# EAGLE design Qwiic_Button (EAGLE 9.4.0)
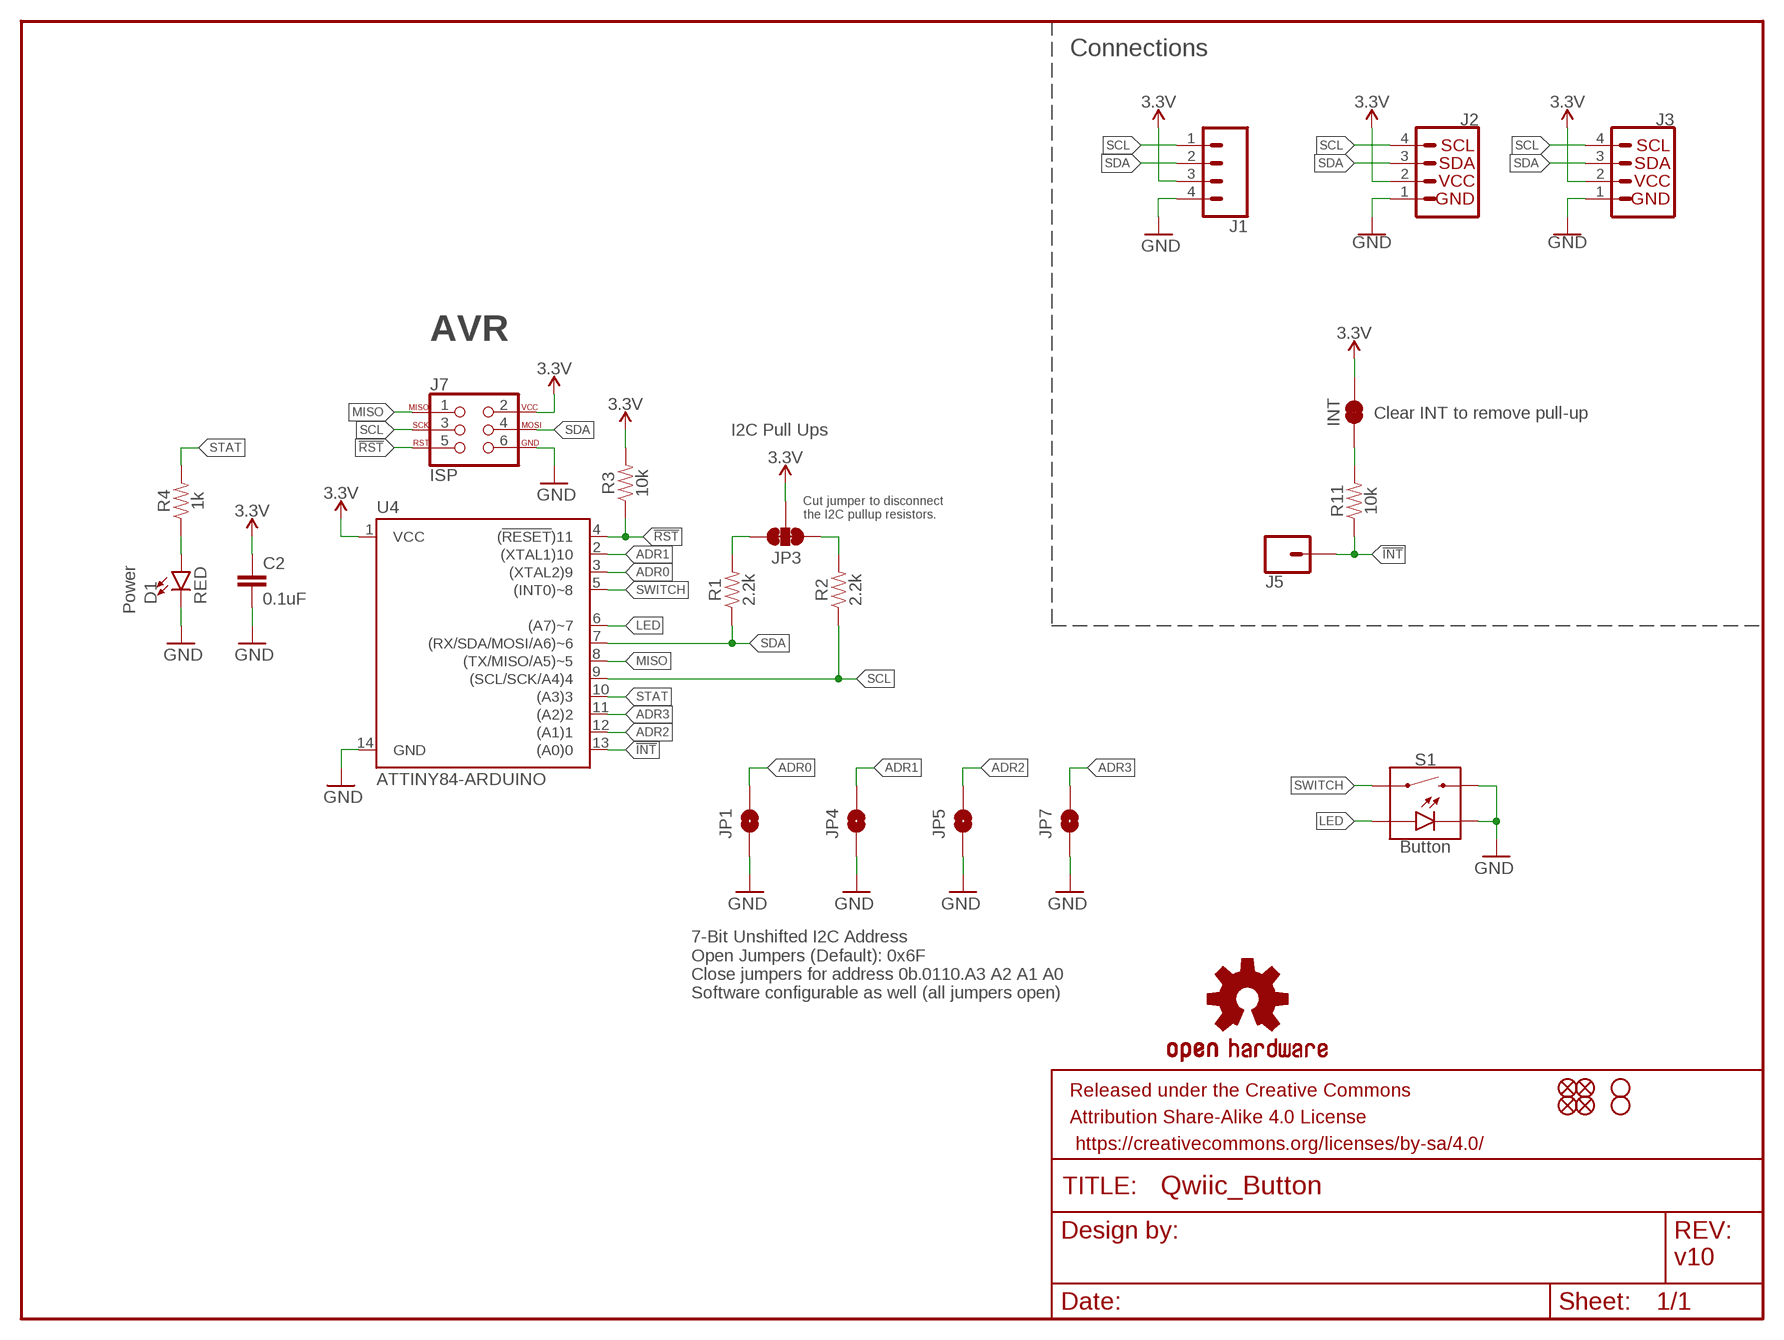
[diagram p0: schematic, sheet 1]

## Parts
C2  0.1uF  0.1UF-0603-25V-(+80/-20%)  [0603]
D1  RED  LED-RED0603  [LED-0603]
FRAME1  FRAME-LETTER  [CREATIVE_COMMONS]
H1  STAND-OFF  [STAND-OFF]
H2  STAND-OFF  [STAND-OFF]
INT  JUMPER-SMT_2_NC_TRACE_SILK  [SMT-JUMPER_2_NC_TRACE_SILK]
J1  CONN_041X04_NO_SILK  [1X04_NO_SILK]
J2  QWIIC_CONNECTORJS-1MM  [JST04_1MM_RA]
J3  QWIIC_CONNECTORJS-1MM  [JST04_1MM_RA]
J5  CONN_01PTH_NO_SILK_YES_STOP  [1X01_NO_SILK]
J7  ISP  AVR_SPI_PROG_3X2TESTPOINTS  [2X3_TEST_POINTS]
JP1  JUMPER-SMT_2_NO_SILK  [SMT-JUMPER_2_NO_SILK]
JP2  FIDUCIALUFIDUCIAL  [MICRO-FIDUCIAL]
JP3  JUMPER-SMT_3_2-NC_TRACE_SILK  [SMT-JUMPER_3_2-NC_TRACE_SILK]
JP4  JUMPER-SMT_2_NO_SILK  [SMT-JUMPER_2_NO_SILK]
JP5  JUMPER-SMT_2_NO_SILK  [SMT-JUMPER_2_NO_SILK]
JP6  FIDUCIALUFIDUCIAL  [MICRO-FIDUCIAL]
JP7  JUMPER-SMT_2_NO_SILK  [SMT-JUMPER_2_NO_SILK]
JP8  FIDUCIALUFIDUCIAL  [MICRO-FIDUCIAL]
JP9  FIDUCIALUFIDUCIAL  [MICRO-FIDUCIAL]
LOGO1  OSHW-LOGOMINI  [OSHW-LOGO-MINI]
R1  2.2k  2.2KOHM-0603-1/10W-1%  [0603]
R2  2.2k  2.2KOHM-0603-1/10W-1%  [0603]
R3  10k  10KOHM-0603-1/10W-1%  [0603]
R4  1k  1KOHM-0603-1/10W-1%  [0603]
R11  10k  10KOHM-0603-1/10W-1%  [0603]
S1  Button  MOMENTARY-SWITCH-SPST-LED-PTH-12MM  [TACTILE_SWITCH_LED_PTH_12MM]
U4  ATTINY84-ARDUINO  [SO14]

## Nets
3.3V: C2.1 INT.2 J1.3 J2.2 J3.2 J7.2 JP3.2 R3.2 U4.1(VCC)
!INT: J5.1 R11.1 U4.13((A0)0)
!RST: J7.5 R3.1 U4.4((!RESET!)11)
ADR0: JP1.2 U4.3((XTAL2)9)
ADR1: JP4.2 U4.2((XTAL1)10)
ADR2: JP5.2 U4.12((A1)1)
ADR3: JP7.2 U4.11((A2)2)
GND: C2.2 D1.C J1.4 J2.1 J3.1 J7.6 JP1.1 JP4.1 JP5.1 JP7.1 S1.2 S1.C U4.14(GND)
INT_R: INT.1 R11.2
LED: S1.A U4.6((A7)~7)
MISO: J7.1 U4.8((TX/MISO/A5)~5)
N$3: D1.A R4.1
SCL: J1.1 J2.4 J3.4 J7.3 R2.1 U4.9((SCL/SCK/A4)4)
SCL_PU1: JP3.1 R2.2
SDA: J1.2 J2.3 J3.3 J7.4 R1.1 U4.7((RX/SDA/MOSI/A6)~6)
SDA_PU1: JP3.3 R1.2
STAT: R4.2 U4.10((A3)3)
SWITCH: S1.4 U4.5((INT0)~8)

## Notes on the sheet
- Connections
- AVR
- Clear INT to remove pull-up
- I2C Pull Ups
- Cut jumper to disconnect
  the I2C pullup resistors.
- Power
- 7-Bit Unshifted I2C Address
  Open Jumpers (Default): 0x6F
  Close jumpers for address 0b.0110.A3 A2 A1 A0
  Software configurable as well (all jumpers open)
- v10

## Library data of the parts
C2 = SparkFun-Capacitors:0.1UF: 0.1µF ceramic capacitors; PROD_ID: CAP-00810
D1 = SparkFun-LED:LED-RED: Red SMD LED; PROD_ID: DIO-00819
FRAME1 = SparkFun-Aesthetics:FRAME-LETTER: Schematic Frame - Letter
H1 H2 = SparkFun-Hardware:STAND-OFF: Stand Off
INT = SparkFun-Jumpers:JUMPER-SMT_2_NC_TRACE: Normally closed trace jumper
J1 = SparkFun-Connectors:CONN_04: Multi connection point. Often used as Generic Header-pin footprint for 0.1 inch spaced/style header connections On any of the 0.1 inch spaced packages, you can populate with these: Break Away Headers - Straight (PRT-00116) Break Away Male Headers - Right Angle (PRT-00553) Female Headers (PRT-00115)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; PROD_ID: CONN-09696
J2 J3 = SparkFun-Connectors:QWIIC_CONNECTOR: SparkFun I2C Standard Qwiic Connector An SMD 1mm pitch JST connector makes it easy and quick (get it? Qwiic?) to connect I2C devices to each other. The Qwiic system enables fast and solderless connection between popular platforms and various sensors and actuators. We carry 200mm, 100mm, 50mm, and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; PROD_ID: CONN-13694
J5 = SparkFun-Connectors:CONN_01: Single connection point. Often used as Generic Header-pin footprint for 0.1 inch spaced/style header connections
J7 = SparkFun-Connectors:AVR_SPI_PROG_3X2: AVR ISP 6 Pin This is the reduced ISP connector for AVR programming. Common on Arduino. This footprint will take up less PCB space and can be used with a 10-pin to 6-pin adapter such as SKU: BOB-08508 **Special note about "TEST_POINT" package. The stop mask is on the top side, so if you want your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
JP1 JP4 JP5 JP7 = SparkFun-Jumpers:JUMPER-SMT_2_NO: Normally open jumper
JP2 JP6 JP8 JP9 = SparkFun:FIDUCIAL: Fiducial Alignment Points
JP3 = SparkFun-Jumpers:JUMPER-SMT_3_2-NC_TRACE: Normally closed trace jumper (2 of 2 connections) This jumper has a trace between all three pads so they are normally closed (NC). Use a razor knife to open the connection(s). For best results follow the IPC guidelines for cutting traces: Cutout at least 0.063 mm (0.005 in). Remove all loose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
LOGO1 = SparkFun-Aesthetics:OSHW-LOGO: Open-Source Hardware (OSHW) Logo
R1 R2 = SparkFun-Resistors:2.2KOHM: 2.2kΩ resistor; PROD_ID: RES-08272
R3 R11 = SparkFun-Resistors:10KOHM: 10kΩ resistor; PROD_ID: RES-00824
R4 = SparkFun-Resistors:1KOHM: 1kΩ resistor; PROD_ID: RES-07856
S1 = SparkFun-Switches:MOMENTARY-SWITCH-SPST-LED: Momentary Switch (Pushbutton) - SPST - w/ LED Normally-open (NO) SPST momentary switches (buttons, pushbuttons), with a built-in LED. Variants PTH-CHERRY - Cherry MX Switch Cherry MX Keyswitches are top-of-the-line mechanical keyboard switches. They’re satisfyingly “clicky”, reliable up to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; PROD_ID: SWCH-11758; SF_SKU: COM-10442
U4 = SparkFun-IC-Microcontroller:ATTINY84-ARDUINO; PROD_ID: IC-14155

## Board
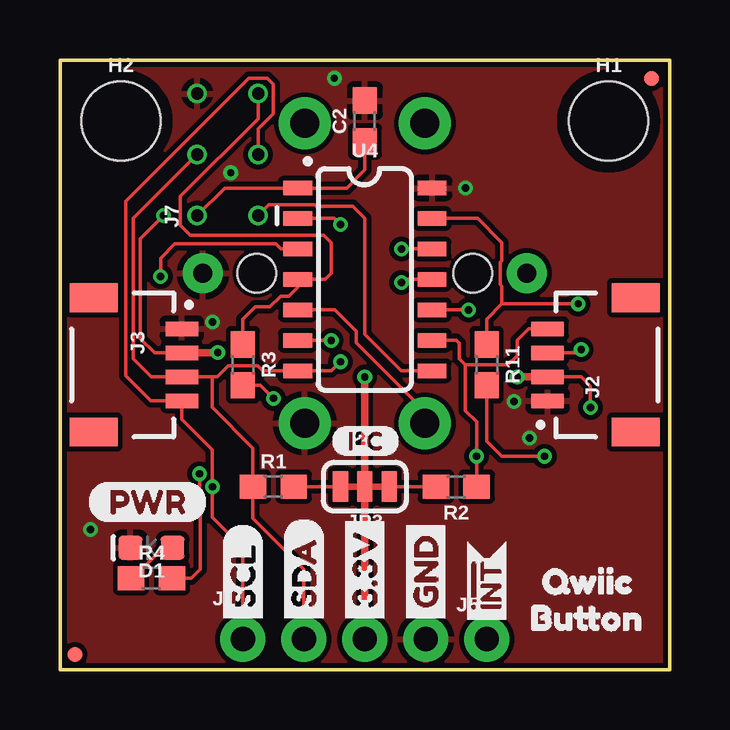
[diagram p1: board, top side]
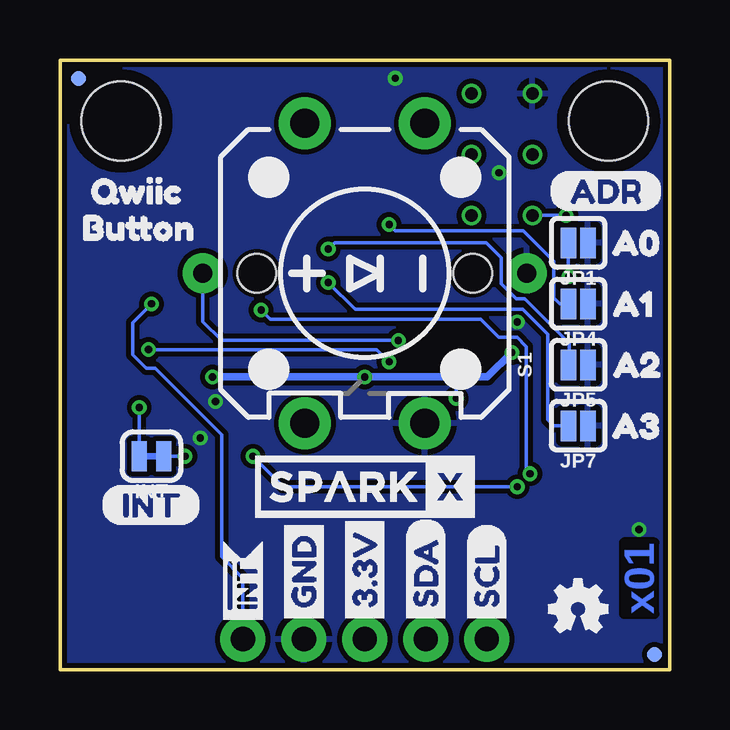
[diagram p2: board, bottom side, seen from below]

Size 25.4 x 25.4 mm. Coordinates in mm from the lower left corner, seen from the top.
Outline: 0,0 25.4,0 25.4,25.4 0,25.4 0,0
Copper layers (1*16): Top 0.035mm / dielectric 1.5mm / Bottom 0.035mm
Design rules "SparkFun-2-layer-PCBWay-LIMIT": minimum track width 6mil, minimum drill 0.3mm, track to track 6mil, track to pad 6mil, pad to pad 6mil, via to via 6mil, smd to smd 6mil, copper to edge 6mil, drill to drill 6mil, minimum pad ring 6mil, minimum via ring 6mil, stop-mask expansion 4mil, vias tented up to drill 25mil, thermal gap 10mil

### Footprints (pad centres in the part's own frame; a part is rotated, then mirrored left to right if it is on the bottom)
0603 = smd 1.1 x 1: 1 -0.85,0; 2 0.85,0
LED-0603 = smd 1 x 1: A -0.877,0; C 0.877,0
STAND-OFF = hole 3.302: 0,0
SMT-JUMPER_2_NC_TRACE_SILK = smd 0.635 x 1.27: 1 -0.508,0; 2 0.508,0
1X04_NO_SILK = drill 1.016 pad 1.88: 1 0,0; 2 2.54,0; 3 5.08,0; 4 7.62,0
JST04_1MM_RA = smd 0.6 x 1.35: 1 -1.5,0; 2 -0.5,0; 3 0.5,0; 4 1.5,0 | smd 1.2 x 2: NC1 2.8,-3.675; NC2 -2.8,-3.675
1X01_NO_SILK = drill 1.016 pad 1.88: 1 0,0
2X3_TEST_POINTS = drill 0.508: 1 -2.54,-1.27; 2 -2.54,1.27; 3 0,-1.27; 4 0,1.27; 5 2.54,-1.27; 6 2.54,1.27
SMT-JUMPER_2_NO_SILK = smd 0.635 x 1.27: 1 -0.406,0; 2 0.406,0
MICRO-FIDUCIAL = smd 0.635 x 0.635: 1 0,0
SMT-JUMPER_3_2-NC_TRACE_SILK = smd 0.635 x 1.27: 1 -1.016,0; 2 0,0; 3 1.016,0
TACTILE_SWITCH_LED_PTH_12MM = drill 1.2 pad 2.159: 1 -6.25,2.5; 2 6.25,2.5; 3 -6.25,-2.5; 4 6.25,-2.5 | drill 0.8 pad 1.676: A 0,-6.75; C 0,6.75 | hole 1.6: 0,4.5; 0,-4.5
SO14 = smd 0.6 x 1.2: 1 -3.175,-2.8; 2 -1.905,-2.8; 3 -0.635,-2.8; 4 0.635,-2.8; 5 1.905,-2.8; 6 3.175,-2.8; 7 4.445,-2.8; 8 4.445,2.8; 9 3.175,2.8; 10 1.905,2.8; 11 0.635,2.8; 12 -0.635,2.8; 13 -1.905,2.8; 14 -3.175,2.8

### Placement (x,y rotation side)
C2  12.7,22.86 90 top
D1  3.81,5.08 180 top
FRAME1  not placed on the board
H1  22.86,22.86 0 top
H2  2.54,22.86 0 top
INT  21.59,8.89 180 bottom
J1  7.62,1.27 0 top
J2  20.32,12.7 90 top
J3  5.08,12.7 270 top
J5  17.78,1.27 0 top
J7  6.99,21.46 90 top
JP1  3.81,17.78 180 bottom
JP2  24.64,24.64 0 bottom
JP3  12.7,7.62 180 top
JP4  3.81,15.24 180 bottom
JP5  3.81,12.7 180 bottom
JP6  0.64,0.64 0 bottom
JP7  3.81,10.16 180 bottom
JP8  0.64,0.64 0 top
JP9  24.64,24.64 0 top
LOGO1  3.81,2.54 0 bottom
R1  8.89,7.62 0 top
R2  16.51,7.62 180 top
R3  7.62,12.7 270 top
R4  3.81,3.81 0 top
R11  17.78,12.7 270 top
S1  12.7,16.51 270 bottom
U4  12.7,16.89 270 top
U$1  [BUTTON1]  18.67,2.16 0 top
U$2  [BUTTON1]  25.4,18.41 0 bottom
U$3  [PWR-()-04]  1.14,6.99 0 top
U$4  [INT-()-04]  23.75,6.86 0 bottom
U$5  [SCL]  7.62,1.65 90 bottom
U$6  [SDA]  10.16,1.65 90 bottom
U$7  [3.3V]  12.7,1.65 90 bottom
U$8  [GND]  15.24,1.65 90 bottom
U$9  [(ADR)]  5.08,19.94 0 bottom
U$10  [I_SUPER2_C-()-03]  11.3,9.53 0 top
U$11  [INT#-[<-04]  17.78,1.4 90 top
U$12  [SDA]  10.16,1.65 90 top
U$13  [GND]  15.24,1.65 90 top
U$14  [SCL]  7.62,1.65 90 top
U$15  [INT#-[<-04]  17.78,1.4 90 bottom
U$16  [A00]  3.3,17.78 0 bottom
U$17  [A11]  3.43,15.24 0 bottom
U$18  [SPARKX-MEDIUM]  12.7,7.62 0 bottom
U$19  [A22]  3.43,12.7 0 bottom
U$20  [QWIIC0]  25.02,19.94 0 bottom
U$21  [A33]  3.3,10.16 0 bottom
U$22  [3.3V]  12.7,1.65 90 top
U$23  [QWIIC0]  19.18,3.68 0 top

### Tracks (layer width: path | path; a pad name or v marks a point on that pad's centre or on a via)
3.3V  (via drill 0.3)
  Top 0.152: J7.2 6.86,20.07 U4.1 11.94,20.07 12.7,20.83 C2.1 | v19.06,12.2 v19.05,12.19 | v6.57,13.21 v6.57,13.2 | R3.2 8.34,11.85 v8.89,11.3 | v22.1,10.92 22.1,11.81 21.71,12.2 J2.2 | J3.2 3.94,13.2 3.35,13.79 3.35,17.96 v4.32,18.92
  Top 0.305: J2.2 v19.06,12.2 | v6.57,13.2 J3.2 | v12.7,12.19 JP3.2 J1.3
  Bottom 0.152: v8.89,11.3 8.89,12.19 | INT.2 v22.1,10.92 | J7.2 v4.32,18.92
  Bottom 0.305: v19.05,12.19 v12.7,12.19 8.89,12.19 7.59,12.19 v6.57,13.21
!INT  (via drill 0.3)
  Top 0.152: U4.13 17.4,18.8 18.41,17.78 18.41,17.04 18.34,16.97 18.34,16.05 18.41,15.98 18.41,15.24 | 18.41,15.24 17.78,14.61 R11.1 | v21.59,15.24 18.41,15.24
  Bottom 0.152: J5.1 17.78,3.81 18.67,4.7 18.67,9.78 21.44,12.55 21.81,12.55 22.38,13.11 22.38,14.45 v21.59,15.23 v21.59,15.24
!RST
  Top 0.152: J7.5 8.26,22.96 5.02,19.72 5.02,18.51 5.43,18.09 10.99,18.09 11.3,17.78 11.3,16.51 11.05,16.26 U4.4 | U4.4 | R3.1 7.62,14.61 8.13,15.11 8.75,15.11 9.19,15.55 9.53,15.55 9.91,15.93 U4.4
ADR0  (via drill 0.3)
  Top 0.152: v4.19,16.38 4.19,17.14 4.79,17.74 8.98,17.74 9.2,17.53 U4.3
  Bottom 0.152: JP1.2 4.22,16.41 v4.19,16.38
ADR1  (via drill 0.3)
  Top 0.152: U4.2 11.43,18.8 v11.68,18.54
  Bottom 0.152: v11.68,18.54 11.43,18.29 6.1,18.29 4.83,17.02 4.83,15.49 4.57,15.24 JP4.2
ADR2  (via drill 0.3)
  Top 0.152: U4.12 v14.22,17.53
  Bottom 0.152: v14.22,17.53 13.96,17.79 7.65,17.79 7.02,17.16 7.02,16.07 6.39,15.44 6.04,15.44 4.19,13.59 4.19,12.72 JP5.2
ADR3  (via drill 0.3)
  Top 0.152: U4.11 14.35,16.26 v14.22,16.13
  Bottom 0.152: v14.22,16.13 13.11,15.01 6.12,15.01 5.08,13.97 5.08,10.41 4.83,10.16 JP7.2
GND  (via drill 0.3)
  other vias: 1.27,5.84 18.92,11.18 19.56,9.65 16.89,20.07 11.43,24.64 6.35,14.48 7.11,20.7
  pour Top (isolate 0.203): 0,0 0,25.4 25.4,25.4 25.4,0
  pour Bottom (isolate 0.203): 0,0 25.4,0 25.4,25.4 0,25.4
INT_R  (via drill 0.3)
  Top 0.152: R11.2 17.78,9.53 18.41,8.89 v20.19,8.89
  Bottom 0.152: v20.19,8.89 INT.1
LED  (via drill 0.3)
  Top 0.152: U4.6 v11.3,13.72
  Bottom 0.152: v11.3,13.72 18.67,13.72 19.45,14.5 S1.A
MISO
  Top 0.152: J7.1 8.7,19.36 10.61,19.36 10.67,19.3 12.19,19.3 12.7,18.8 12.7,13.97 14.22,12.45 U4.8
N$3
  Top 0.152: R4.1 3.04,3.81 4.31,5.08 D1.A
SCL  (via drill 0.3)
  Top 0.152: U4.9 16.51,13.72 16.64,13.59 16.64,12.95 16.89,12.7 | 16.89,12.7 18.66,12.7 18.79,12.83 18.8,12.83 19.05,13.08 19.05,13.72 19.53,14.2 J2.4 | R2.1 v17.36,8.89 17.36,10.33 16.89,10.79 16.89,12.7 | J1.1 7.62,5.08 6.35,6.35 v6.35,7.62 6.35,9.17 5.08,10.44 J3.4 3.79,11.2 2.74,12.24 2.74,19.52 7.87,24.64 8.64,24.64 8.89,24.39 8.89,23.16 8.26,22.53 J7.3
  Bottom 0.152: v6.35,7.62 16.09,7.62 v17.36,8.89
SCL_PU1
  Top 0.152: JP3.1 R2.2
SDA  (via drill 0.3)
  Top 0.152: J7.4 3.05,18.8 3.05,12.95 3.8,12.2 J3.3 6.35,12.2 | 6.35,12.2 6.54,12.2 7.01,12.67 8.23,12.67 8.45,12.45 U4.7 11.3,12.45 v11.68,12.83 | J1.2 10.16,4.19 8.04,6.31 R1.1 8.04,9.23 6.35,10.92 6.35,12.2 | J2.3 21.58,13.2 v21.72,13.34
  Bottom 0.152: v21.72,13.34 12.19,13.34 v11.68,12.83
SDA_PU1
  Top 0.152: JP3.3 R1.2
STAT  (via drill 0.3)
  Top 0.152: R4.2 5.46,3.81 5.84,4.19 5.84,7.37 5.82,7.4 5.82,7.84 5.84,7.87 5.84,8.13 v5.81,8.16 | v17.02,14.99 U4.10
  Bottom 0.152: v17.02,14.99 16.64,14.61 7.87,14.61 7.11,13.84 6.35,13.84 5.97,13.46 5.97,8.32 v5.81,8.16
SWITCH
  Top 0.152: S1.4 15.2,10.77 12.34,13.62 12.34,14.1 11.46,14.99 U4.5

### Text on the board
Bottom: x01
